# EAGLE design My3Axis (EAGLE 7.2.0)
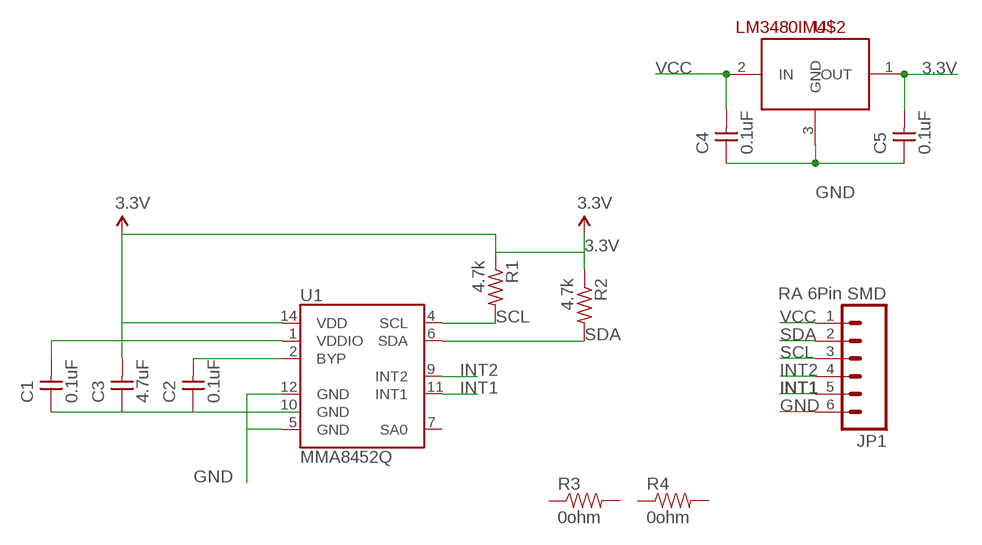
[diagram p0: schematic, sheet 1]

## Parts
C1  0.1uF  UNPOLARIZED_CAPACITOR1206  [1206]
C2  0.1uF  UNPOLARIZED_CAPACITOR1206  [1206]
C3  4.7uF  UNPOLARIZED_CAPACITOR1206  [1206]
C4  0.1uF  UNPOLARIZED_CAPACITOR1206  [1206]
C5  0.1uF  UNPOLARIZED_CAPACITOR1206  [1206]
JP1  RA 6Pin SMD  M06SMD  [1X06-SMD]
R1  4.7k  RESISTOR1206  [1206]
R2  4.7k  RESISTOR1206  [1206]
R3  0ohm  RESISTOR1206  [1206]
R4  0ohm  RESISTOR1206  [1206]
U1  MMA8452Q  [QFN-16_0.5MM]
U$2  LM3480IM4  [SOT23-3]

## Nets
3.3V: C1.2 C3.2 C5.2 R1.1 R2.1 U1.1(VDDIO) U$2.1(OUT)
BYP: C2.2 U1.2(BYP)
GND: C1.1 C2.1 C3.1 C4.1 C5.1 JP1.6 U1.12(GND) U$2.3(GND)
INT1: JP1.5 U1.11(INT1)
INT2: JP1.4 U1.9(INT2)
N$3: U1.5(GND)
N$4: U1.14(VDD)
SCL: JP1.3 R1.2 U1.4(SCL)
SDA: JP1.2 R2.2 U1.6(SDA)
VCC: C4.2 JP1.1 U$2.2(IN)
Unconnected: R3.1 R3.2 R4.1 R4.2 U1.7(SA0) U1.10(GND)

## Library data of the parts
C1-C5 = ng:UNPOLARIZED_CAPACITOR: unpolarized_capacitor
JP1 = SparkFun-Connectors:M06: Header 6 Standard 6-pin 0.1" header. Use with straight break away headers (SKU : PRT-00116), right angle break away headers (PRT-00553), swiss pins (PRT-00743), machine pins (PRT-00117), and female headers (PRT-00115). Molex polarized connector foot print use with SKU : PRT-08094 with associated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; PROD_ID: CONN-08971
R1 R2 = ng:RESISTOR
R3 R4 = SparkFun-Resistors:RESISTOR: Resistor
U1 = SparkFun-Sensors:MMA8452Q: MMA8452Q 3-Axis, 12/8-bit Digital Accelerometer Supply Voltage: 1.6-3.6V Range: +/- 2g, 4g, 8g Interface: I2C, 12-bit and 8-bit ODR: 1.56 Hz - 800 Hz Package: QFN-16 http://cache.freescale.com/files/sensors/doc/data_sheet/MMA8452Q.pdf; PROD_ID: IC-10769
U$2 = SparkFun-PowerIC:LM3480IM4: Small package linear regulator

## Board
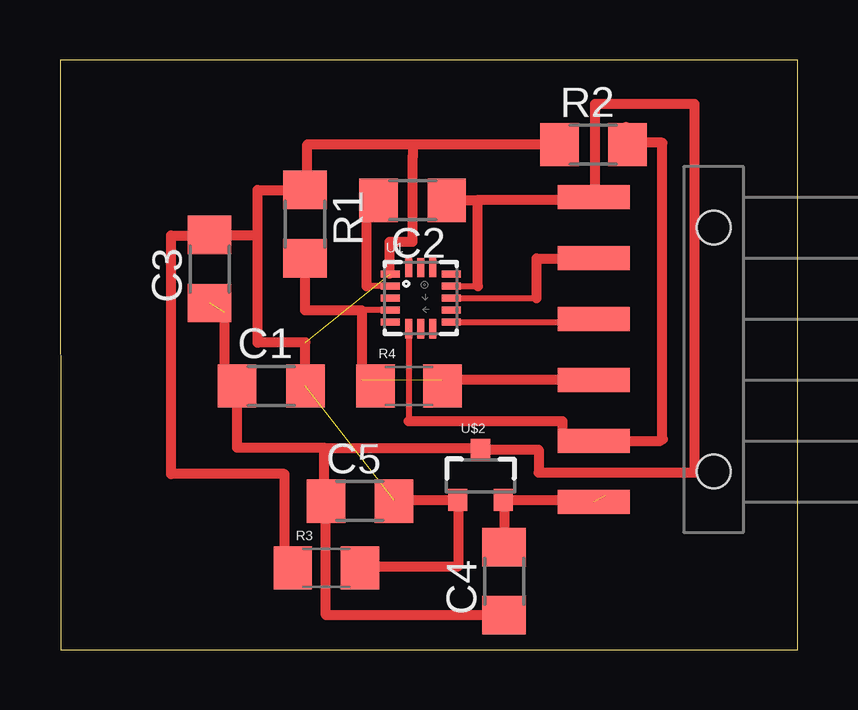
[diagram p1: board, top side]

Size 30.75 x 24.59 mm. Coordinates in mm from the lower left corner, seen from the top.
Outline: 0.03,0 30.75,0 30.73,24.59 0,24.59 0.03,0
Copper layers (1*16): Top 0.035mm / dielectric 1.5mm / Bottom 0.035mm
Design rules "default": minimum track width 10mil, minimum drill 24mil, track to track 8mil, track to pad 8mil, pad to pad 8mil, via to via 8mil, smd to smd 8mil, copper to edge 40mil, drill to drill 8mil, minimum pad ring 10mil, minimum via ring 8mil, stop-mask expansion 4mil, vias tented up to drill 0mil, thermal gap 10mil

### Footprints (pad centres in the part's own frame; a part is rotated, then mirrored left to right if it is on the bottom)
1206 = smd 1.6 x 1.803: 1 -1.422,0; 2 1.422,0
1X06-SMD = smd 1 x 3: 1 -6.35,5; 2 -3.81,5; 3 -1.27,5; 4 1.27,5; 5 3.81,5; 6 6.35,5 | hole 1.4: -5.08,0; 5.08,0
1206' = smd 1.6 x 1.8: 1 -1.4,0; 2 1.4,0
QFN-16_0.5MM = smd 0.8 x 0.3: 1 -1.275,1; 2 -1.275,0.5; 3 -1.275,0; 4 -1.275,-0.5; 5 -1.275,-1; 9 1.275,-1; 10 1.275,-0.5; 11 1.275,0; 12 1.275,0.5; 13 1.275,1 | smd 0.3 x 0.8: 6 -0.5,-1.275; 7 0,-1.275; 8 0.5,-1.275; 14 0.5,1.275; 15 0,1.275; 16 -0.5,1.275
SOT23-3 = smd 0.8 x 0.9: 1 -0.95,-1; 2 0.95,-1; 3 0,1.1

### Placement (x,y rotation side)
C1  8.8,11 0 top
C2  14.69,18.74 180 top
C3  6.23,15.88 90 top
C4  18.5,2.86 90 top
C5  12.5,6.2 0 top
JP1  27.24,12.52 90 top
R1  10.21,17.75 270 top
R2  22.23,21.06 0 top
R3  0ohm  [1206']  11.1,3.41 0 top
R4  0ohm  [1206']  14.54,11 0 top
U1  15.03,14.66 0 top
U$2  17.52,7.25 0 top

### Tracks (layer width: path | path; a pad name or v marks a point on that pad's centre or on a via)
3.3V  (2 unrouted)
  Top 0.406: U$2.1 16.68,6.25 16.68,6.22 13.92,6.22 C5.2 | C1.2 10.23,12.82 8.25,12.82 8.25,12.81 8.24,12.81 8.24,17.3 | R2.1 14.69,21.06 | 14.69,21.06 14.69,20.51 | 14.69,21.06 14.69,21.07 10.31,21.07 10.31,19.17 R1.1 8.24,19.17 8.24,17.62 8.24,17.3 | C3.2 8.24,17.3
BYP
  Top 0.254: U1.2 12.77,15.16
  Top 0.406: 12.77,15.16 12.77,18.86 12.77,18.88 C2.2
GND  (1 unrouted)
  Top 0.254: U1.12 17.42,15.16
  Top 0.406: 22.24,18.8 JP1.6 | 26.45,7.39 19.94,7.39 19.94,8.35 U$2.3 17.52,8.42 11,8.42 | 17.42,15.16 17.42,18.74 | JP1.6 22.24,18.84 21.34,18.84 21.34,18.77 17.42,18.77 17.42,18.74 | C2.1 17.42,18.74 | 11,8.42 11,6.2 C5.1 11.08,1.44 C4.1 | 11,8.42 7.38,8.42 C1.1 6.86,11 6.86,14.05 | JP1.6 22.3,18.87 22.3,22.75 26.45,22.75 26.45,7.39 | 26.47,7.39 26.45,7.39
INT1
  Top 0.254: U1.11 19.86,14.66
  Top 0.406: JP1.5 22.24,16.3 21.71,16.3 21.71,16.32 19.86,16.32 19.86,14.8 19.86,14.66
INT2
  Top 0.254: U1.9 21.64,13.66
  Top 0.406: 22.86,13.85 22.86,13.66 21.64,13.66 21.64,13.79 JP1.4
N$1
  Top 0.406: 12.84,3.48 16.61,3.48 16.61,6.07
N$5
  Top 0.406: 13.74,15.68 13.74,17.02 14.69,17.02 14.69,17.03 14.69,20.56
N$7
  Top 0.406: 9.32,3.94 9.36,3.94 9.36,7.33 4.63,7.33 4.63,17.28 5.94,17.28 5.94,17.32
SCL  (1 unrouted)
  Top 0.254: U1.4 12.57,14.16
  Top 0.406: JP1.3 15.9,11.25 15.9,11.24 | R1.2 10.2,14.16 12.57,14.16 12.57,11.27
SDA  (1 unrouted)
  Top 0.254: U1.6 14.52,9.53
  Top 0.406: 25.1,8.79 25.03,8.79 25.03,8.71 JP1.2 22.24,8.79 20.94,8.79 20.94,9.53 14.52,9.53 | 23.59,21.8 R2.2 23.65,21.13 25.1,21.13 25.1,8.79 | 25.13,8.79 25.1,8.79
VCC  (1 unrouted)
  Top 0.406: 22.14,6.14 JP1.1 | C4.2 18.5,6.25 U$2.2 22.72,6.25 22.72,6.41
